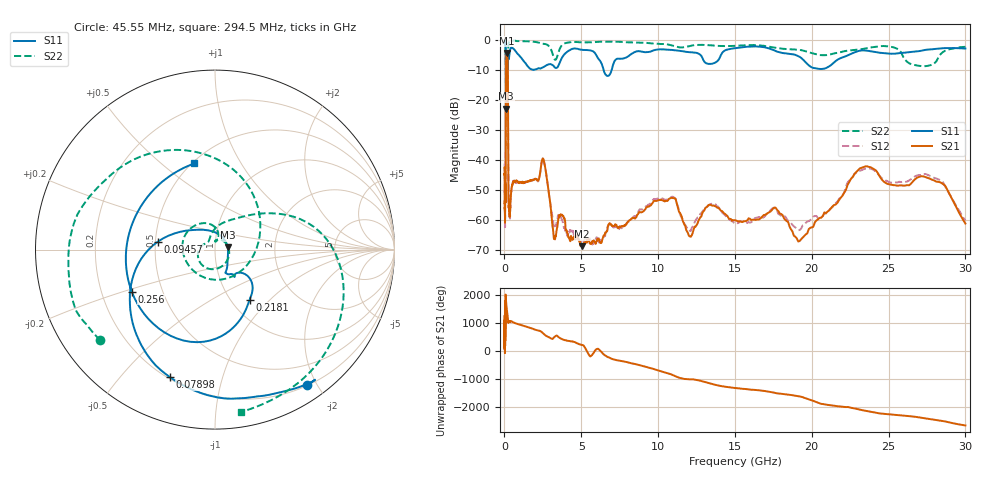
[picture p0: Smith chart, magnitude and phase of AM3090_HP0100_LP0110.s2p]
! Date/Time: Thu, Feb 28, 2019 1:57 PM
! Network Analyzer: Agilent Technologies E8364B Rev: A.07.50.67
! Sweep from 0.010 to 30.000 GHz, 1601 Points, Sweep Type: LOG
! Power Supply: 5.023 V, 0.002 A
# Hz S DB R 50
!freq MagS11 AngS11 MagS21 AngS21 MagS12 AngS12 MagS22 AngS22
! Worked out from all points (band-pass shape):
!   1601 points, 10 MHz to 30 GHz, reference 50 ohm
!   highest |S21| = -4.38 dB at 152.9 MHz (marker M1); lowest = -68.8 dB at 5.052 GHz (marker M2)
!   |S21| within 3 dB of the highest: 105.6 MHz to 210.9 MHz (105.3 MHz wide, 66.5 % of centre)
!   lowest |S11| = -22.9 dB at 103.5 MHz (marker M3), VSWR 1.15, Z = 57.6 + j1.43 ohm
!   |S11| at or under -10 dB: 94.66 MHz to 213.5 MHz (118.8 MHz wide, 77.1 % of centre); 6.455 GHz to 6.979 GHz (524.3 MHz wide, 7.81 % of centre)
!   |S22| runs from -27.0 to -0.2 dB; largest |S21 - S12| = 0.013
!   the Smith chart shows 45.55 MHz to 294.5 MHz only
!   S11 on the Smith chart (normalised r, x): 45.55 MHz: 0.21, -1.88; 78.98 MHz: 0.21, -0.69; 94.57 MHz: 0.52, +0.05; 218.1 MHz: 1.21, -0.77; 256 MHz: 0.33, -0.21; 294.5 MHz: 0.51, +0.65
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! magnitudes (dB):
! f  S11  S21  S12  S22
! 10 MHz  -0.2  -42.5  -41.2  -0.6
! 38.04 MHz  -0.5  -59.8  -59.9  -1.4
! 45.55 MHz  -0.8  -51.8  -54.4  -1.8
! 78.98 MHz  -2.5  -48.4  -47.9  -4.7
! 94.57 MHz  -9.9  -16.8  -16.9  -15.3
! 103.5 MHz  -22.9  -8.2  -8.2  -14.7
! 144.7 MHz  -15.9  -4.4  -4.4  -23.1
! 152.9 MHz  -15.6  -4.4  -4.3  -21.3
! 196.4 MHz  -14.0  -5.6  -5.6  -24.8
! 218.1 MHz  -9.4  -9.2  -9.2  -13.9
! 256 MHz  -5.7  -48.8  -49.9  -1.8
! 294.5 MHz  -6.1  -56.7  -56.8  -0.8
! 550.5 MHz  -2.8  -47.6  -47.4  -0.3
! 2.084 GHz  -9.8  -46.5  -46.5  -0.7
! 2.533 GHz  -9.0  -39.7  -39.7  -1.3
! 3.236 GHz  -8.9  -66.3  -62.3  -6.2
! 5.052 GHz  -3.3  -68.8  -67.0  -0.8
! 7.926 GHz  -5.8  -61.6  -61.3  -0.8
! 10.7 GHz  -3.3  -53.0  -52.9  -1.6
! 19.31 GHz  -6.0  -66.4  -62.9  -3.4
! 23.48 GHz  -3.5  -42.2  -42.9  -2.9
! 30 GHz  -2.9  -61.2  -60.2  -2.3
